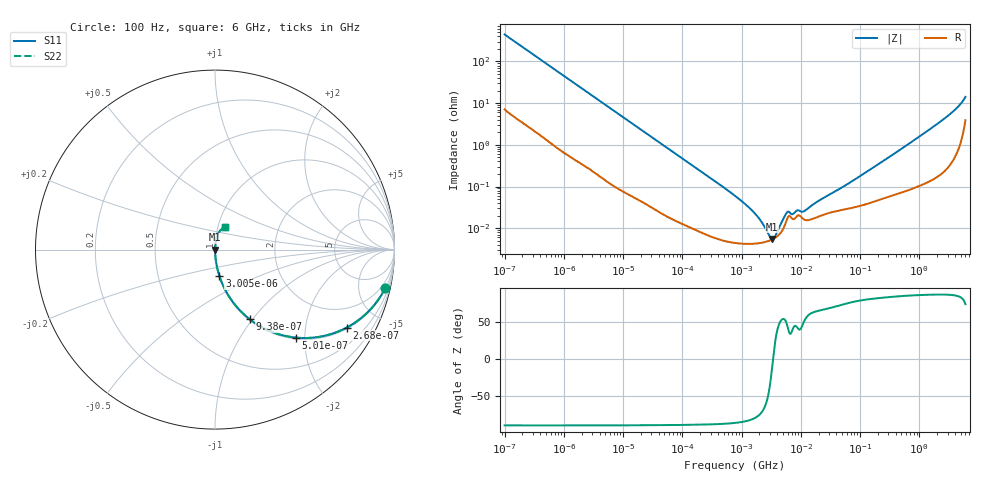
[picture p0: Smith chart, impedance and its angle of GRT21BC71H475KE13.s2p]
!Murata Part Number: GRT21BC71H475KE13
!These Parameters are Measured in Series Mode Connection
!Data Generated on Jun 19, 2026
!  o--ll--o
!Port1  Port2
!  o------o
!Operation Temp=25[degC], DC Bias Voltage=0[V]
!Freq. Start=100[Hz] Stop=6[GHz] 401[Steps]
# Hz S RI R 50
!Freq.(Hz) S11(Real) S11(Imag) S21(Real) S21(Imag) S12(Real) S12(Imag) S22(Real) S22(Imag)
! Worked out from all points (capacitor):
!   401 points, 100 Hz to 6 GHz, reference 50 ohm
!   read as one part in series: C = 3.57 uF near 109 Hz
!   lowest |Z| = 5.48 mohm at 3.246 MHz (marker M1)
!   series resonance near 3.392 MHz, so ESL is about 620 pH
!   S11 on the Smith chart (normalised r, x): 100 Hz: 1.14, -8.90; 268 Hz: 1.05, -3.35; 501 Hz: 1.03, -1.80; 938 Hz: 1.01, -0.97; 3.005 kHz: 1.00, -0.31; 6 GHz: 1.08, +0.27
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100  0.9489 -0.2125  0.0511 0.2125  0.0511 0.2125  0.9489 -0.2125
164  0.878 -0.3198  0.122 0.3198  0.122 0.3198  0.878 -0.3198
268  0.7342 -0.4342  0.2658 0.4342  0.2658 0.4342  0.7342 -0.4342
501  0.4488 -0.4901  0.5512 0.4901  0.5512 0.4901  0.4488 -0.4901
938  0.1931 -0.3877  0.8069 0.3877  0.8069 0.3877  0.1931 -0.3877
2008  0.0522 -0.2149  0.9478 0.2149  0.9478 0.2149  0.0522 -0.2149
3005  0.025 -0.1485  0.975 0.1485  0.975 0.1485  0.025 -0.1485
8801  0.00359 -0.0524  0.9964 0.0524  0.9964 0.0524  0.00359 -0.0524
40335  0.000381 -0.0117  0.9996 0.0117  0.9996 0.0117  0.000381 -0.0117
774597  4.45e-05 -0.000598  1 0.000598  1 0.000598  4.45e-05 -0.000598
1516199  4.23e-05 -0.00026  1 0.00026  1 0.00026  4.23e-05 -0.00026
2481164  4.66e-05 -9.38e-05  1 9.38e-05  1 9.38e-05  4.66e-05 -9.38e-05
3245845  5.32e-05 -1.33e-05  0.9999 1.33e-05  0.9999 1.33e-05  5.32e-05 -1.33e-05
4246196  6.89e-05 7.13e-05  0.9999 -7.13e-05  0.9999 -7.13e-05  6.89e-05 7.13e-05
5554849  0.000134 0.000168  0.9999 -0.000168  0.9999 -0.000168  0.000134 0.000168
6075234  0.000188 0.000166  0.9998 -0.000166  0.9998 -0.000166  0.000188 0.000166
1.137099e7  0.000161 0.000198  0.9998 -0.000198  0.9998 -0.000198  0.000161 0.000198
1.555665e7  0.000166 0.000318  0.9998 -0.000318  0.9998 -0.000318  0.000166 0.000318
3.124326e8  0.000601 0.0051  0.9994 -0.0051  0.9994 -0.0051  0.000601 0.0051
2.679998e9  0.00418 0.0429  0.9958 -0.0429  0.9958 -0.0429  0.00418 0.0429
4.193612e9  0.0111 0.0724  0.9889 -0.0724  0.9889 -0.0724  0.0111 0.0724
6e9  0.0536 0.1239  0.9464 -0.1239  0.9464 -0.1239  0.0536 0.1239
